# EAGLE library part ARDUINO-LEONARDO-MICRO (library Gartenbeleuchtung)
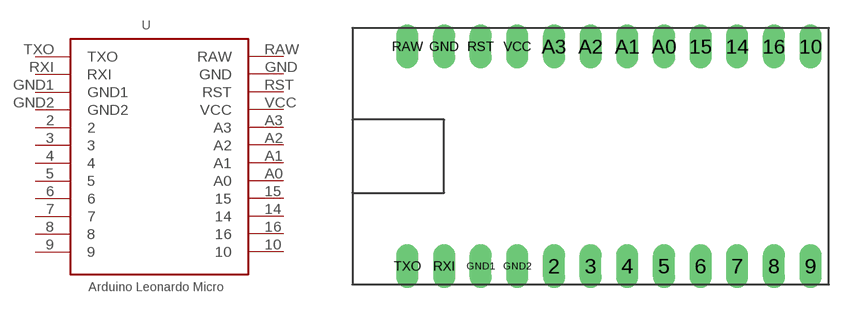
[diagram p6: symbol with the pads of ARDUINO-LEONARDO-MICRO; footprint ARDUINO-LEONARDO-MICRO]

Designator prefix -

## ARDUINO-LEONARDO-MICRO  [ARDUINO-LEONARDO-MICRO]
2  2
3  3
4  4
5  5
6  6
7  7
8  8
9  9
10  10
14  14
15  15
16  16
A0  A0
A1  A1  pwr
A2  A2
A3  A3
GND  GND  pwr
GND1  GND1  pwr
GND2  GND2  pwr
RAW  RAW
RST  RST
RXI  RXI
TXO  TXO
VCC  VCC  pwr

## Footprint ARDUINO-LEONARDO-MICRO (pad centres in mm)
drill 1 pad 1.422 long: 2 10.16,0; 3 12.7,0; 4 15.24,0; 5 17.78,0; 6 20.32,0; 7 22.86,0; 8 25.4,0; 9 27.94,0; 10 27.94,15.24; 14 22.86,15.24; 15 20.32,15.24; 16 25.4,15.24; A0 17.78,15.24; A1 15.24,15.24; A2 12.7,15.24; A3 10.16,15.24; GND 2.54,15.24; GND1 5.08,0; GND2 7.62,0; RAW 0,15.24; RST 5.08,15.24; RXI 2.54,0; TXO 0,0; VCC 7.62,15.24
